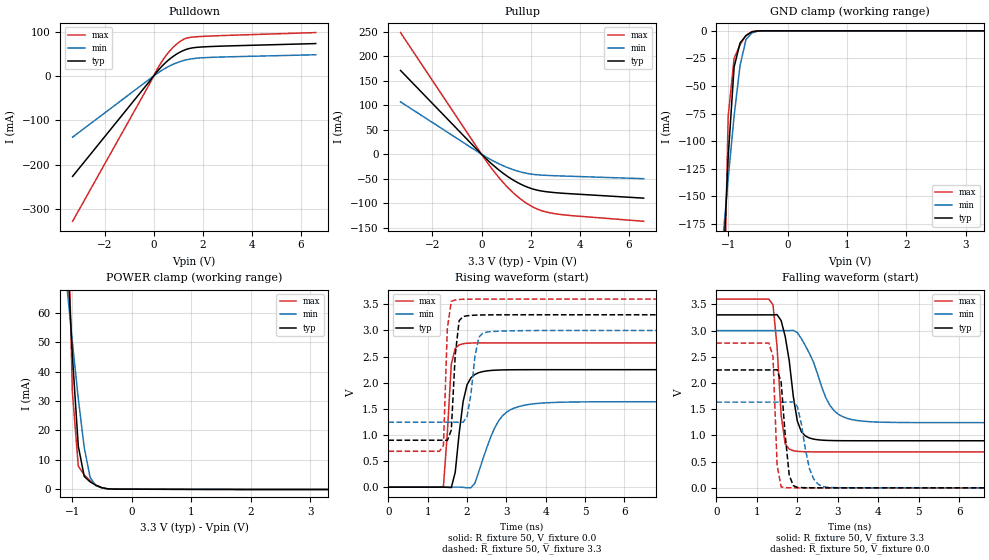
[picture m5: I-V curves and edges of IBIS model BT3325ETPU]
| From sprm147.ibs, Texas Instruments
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[Model]   BT3325ETPU
Model_type   I/O
Vinh = 2.00
Vinl = 0.80
Enable   Active-Low
Polarity   Non-Inverting
| signals   A, GZ, Y
Vmeas = 1.5
|   typ   min   max
C_comp   1.3948367p   1.3632639p   1.426735p
|   typ   min   max
[Temperature Range]   25   -40   125
|   typ   min   max
[Voltage Range]   3.30V   3.00V   3.60V
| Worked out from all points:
|   slope of the pulldown table from 0 to 0.495 V, typ, clamps not added: 16.2 ohm
|   slope of the pullup table from 0 to 0.495 V, typ, clamps not added: 21.2 ohm
|   GND clamp passes 1 mA (typ) near -0.60 V on its own axis
|   POWER clamp passes 1 mA (typ) near -0.56 V on its own axis
|   rising waveform, R_fixture 50, V_fixture 0.0: 20-80 % time 228ps typ, 532ps min, 137ps max; typ from 0 V to 2.25 V
|   falling waveform, R_fixture 50, V_fixture 3.3: 20-80 % time 263ps typ, 547ps min, 162ps max; typ from 3.3 V to 0.899 V
|   rising waveform, R_fixture 50, V_fixture 3.3: 20-80 % time 124ps typ, 184ps min, 77.7ps max; typ from 0.899 V to 3.3 V
|   falling waveform, R_fixture 50, V_fixture 0.0: 20-80 % time 151ps typ, 247ps min, 80.7ps max; typ from 2.25 V to 0 V
[Pulldown]
|   Voltage   I(typ)   I(min)   I(max)
-3.3V     -226mA     -137.8mA   -327.2mA
-200mV    -14.16mA   -8.386mA   -21.14mA
200mV     13.61mA    7.952mA    20.54mA
400mV     25.49mA    15.02mA    38.03mA
600mV     35.71mA    21.19mA    52.74mA
1V        51.44mA    30.9mA     74.72mA
1.3V      59.31mA    35.9mA     84.44mA
1.7V      64.08mA    39.68mA    88.13mA
6.6V      72.96mA    47.76mA    97.72mA
[GND_clamp]
|   Voltage   I(typ)   I(min)   I(max)
-3.3V     -3.509A    -1.717A    -9.214A
-1.1V     -235.6mA   -195.9mA   -329.9mA
-1V       -114.5mA   -134.1mA   -77.56mA
-900mV    -32.77mA   -77.19mA   -24.88mA
-800mV    -11.03mA   -31.34mA   -12.64mA
-700mV    -4.297mA   -7.901mA   -4.239mA
-600mV    -942.8uA   -1.867mA   -603.3uA
-500mV    -96.85uA   -342.9uA   -35.84uA
-400mV    -6.084uA   -43.55uA   -1.084uA
3.3V      222pA      10.71uA    0A
[Pullup]
|   Voltage   I(typ)   I(min)   I(max)
-3.3V     171mA      106.9mA    248.3mA
300mV     -14.55mA   -8.884mA   -21.5mA
700mV     -31.87mA   -19.32mA   -47.22mA
1V        -43.2mA    -26mA      -64.19mA
1.6V      -61.21mA   -36.17mA   -91.8mA
1.9V      -67.72mA   -39.52mA   -102.3mA
2.2V      -72.46mA   -41.63mA   -110.4mA
2.5V      -75.47mA   -42.73mA   -116.1mA
2.9V      -77.9mA    -43.66mA   -120.6mA
3.7V      -80.82mA   -45.04mA   -125.3mA
6.6V      -89.55mA   -49.85mA   -136.8mA
[POWER_clamp]
|   Voltage   I(typ)   I(min)   I(max)
-3.3V     1.144A     573.6mA    2.732A
-1.1V     86.36mA    70.97mA    117.9mA
-1V       45.71mA    50.25mA    33.28mA
-900mV    14.66mA    30.83mA    7.867mA
-800mV    4.346mA    14.17mA    4.834mA
-700mV    2.465mA    3.934mA    2.867mA
-600mV    1.311mA    1.11mA     1.364mA
-500mV    503.7uA    394.3uA    412.6uA
-300mV    29.28uA    25.65uA    34.36uA
3.3V      -100.1uA   -62.39uA   -157uA
[Ramp]
|   I(typ)   I(min)   I(max)
dV/dt_r   1.349/0.218n   0.981/0.527n   1.658/0.107n
dV/dt_f   1.441/0.253n   1.053/0.544n   1.748/0.140n
[Rising Waveform]
R_fixture = 50
V_fixture = 0.0
|  pu_on
|  TIME   V(typ)   V(min)   V(max)
0s        15nV       177nV      1nV
1.4ns     469.7uV    -1.146uV   14.49mV
1.6ns     -7.514mV   -4.324uV   2.355V
1.7ns     285mV      327.9uV    2.656V
1.8ns     1.031V     946.7uV    2.723V
1.9ns     1.637V     -3.679mV   2.746V
2.1ns     2.094V     -9.321mV   2.759V
2.8ns     2.242V     1.266V     2.763V
3.3ns     2.248V     1.539V     2.763V
9.8ns     2.249V     1.636V     2.763V
[Falling Waveform]
R_fixture = 50
V_fixture = 3.3
V_fixture_min = 3.0
V_fixture_max = 3.6
|  pd_on
|  TIME   V(typ)   V(min)   V(max)
0s        3.3V       3V         3.6V
1.4ns     3.299V     3V         3.489V
1.5ns     3.305V     3V         2.694V
1.6ns     3.191V     3V         1.389V
1.7ns     2.889V     2.999V     839.4mV
1.9ns     1.747V     3.005V     709.6mV
2.2ns     989.7mV    2.71V      688.6mV
2.8ns     903.3mV    1.578V     686.1mV
3.3ns     898.9mV    1.31V      686.2mV
10ns      898.6mV    1.244V     686.2mV
[Rising Waveform]
R_fixture = 50
V_fixture = 3.3
V_fixture_min = 3.0
V_fixture_max = 3.6
|  pd_off
|  TIME   V(typ)   V(min)   V(max)
0s        898.6mV    1.244V     686.2mV
1.4ns     898.9mV    1.244V     797.8mV
1.5ns     894.4mV    1.244V     3.049V
1.6ns     1.094V     1.245V     3.558V
1.7ns     2.532V     1.244V     3.585V
1.8ns     3.188V     1.24V      3.593V
1.9ns     3.266V     1.243V     3.597V
2.3ns     3.295V     2.867V     3.6V
2.4ns     3.297V     2.949V     3.6V
10ns      3.3V       3V         3.6V
[Falling Waveform]
R_fixture = 50
V_fixture = 0.0
|  pu_off
|  TIME   V(typ)   V(min)   V(max)
0s        2.249V     1.636V     2.763V
1.3ns     2.249V     1.636V     2.763V
1.4ns     2.248V     1.636V     2.498V
1.5ns     2.254V     1.635V     444.9mV
1.6ns     2.02V      1.635V     17.03mV
1.8ns     240.6mV    1.637V     2.275mV
2ns       9.578mV    1.553V     611.2uV
2.3ns     1.589mV    363.8mV    125.2uV
2.6ns     409.9uV    33.25mV    46.62uV
10ns      1.581uV    1.085uV    134nV
